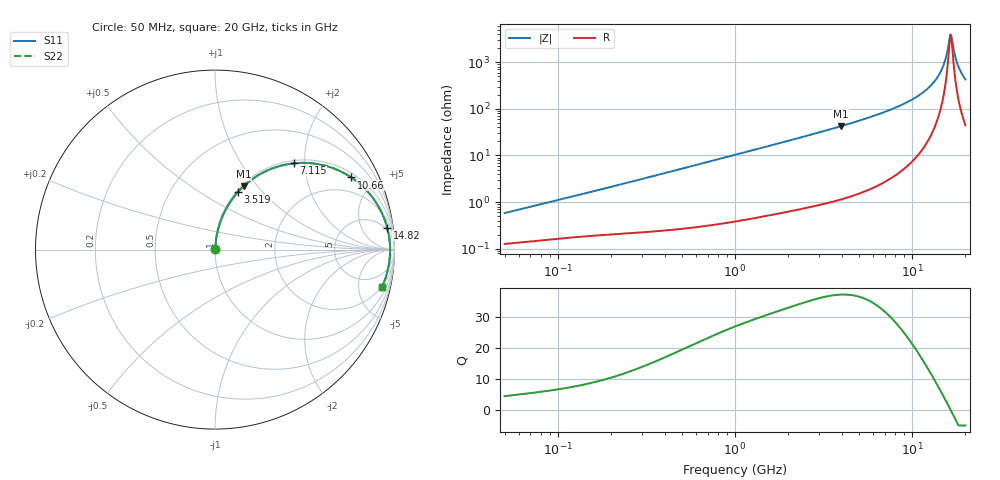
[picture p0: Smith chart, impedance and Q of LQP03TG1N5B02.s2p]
!Murata Part Number: LQP03TG1N5B02
!These Parameters are Measured in Series Mode Connection
!  o--[Z]--o
!Port1  Port2
!  o-------o
!Freq. Start=50[MHz] Stop=20[GHz], 401[Steps]
# Hz S RI R 50
!Freq.(Hz) S11(Real) S11(Imag) S21(Real) S21(Imag) S12(Real) S12(Imag) S22(Real) S22(Imag)
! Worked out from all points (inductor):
!   401 points, 50 MHz to 20 GHz, reference 50 ohm
!   read as one part in series: L = 1.78 nH near 51.52 MHz
!   highest Q = 37.3 at 3.967 GHz (marker M1), where L = 1.71 nH
!   self-resonance near 16.46 GHz
!   S11 on the Smith chart (normalised r, x): 50 MHz: 1.00, +0.01; 3.519 GHz: 1.02, +0.75; 7.115 GHz: 1.06, +1.76; 10.66 GHz: 1.19, +3.67; 14.82 GHz: 4, +15; 20 GHz: 1.89, -8.55
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5e7  0.0013 0.00565  0.9987 -0.00565  0.9987 -0.00565  0.0013 0.00565
1.364002e8  0.00203 0.0146  0.998 -0.0146  0.998 -0.0146  0.00203 0.0146
3.721004e8  0.00388 0.0386  0.9961 -0.0386  0.9961 -0.0386  0.00388 0.0386
1e9  0.0142 0.1013  0.9858 -0.1013  0.9858 -0.1013  0.0142 0.1013
2.728004e9  0.081 0.2591  0.919 -0.2591  0.919 -0.2591  0.081 0.2591
3.519108e9  0.1285 0.3215  0.8715 -0.3215  0.8715 -0.3215  0.1285 0.3215
3.967106e9  0.1597 0.3532  0.8403 -0.3532  0.8403 -0.3532  0.1597 0.3532
5.352748e9  0.2721 0.4314  0.7279 -0.4314  0.7279 -0.4314  0.2721 0.4314
7.114996e9  0.4379 0.4805  0.5621 -0.4805  0.5621 -0.4805  0.4379 0.4805
7.442007e9  0.4698 0.4829  0.5302 -0.4829  0.5302 -0.4829  0.4698 0.4829
1.066139e10  0.7596 0.4019  0.2404 -0.4019  0.2404 -0.4019  0.7596 0.4019
1.295331e10  0.8995 0.2592  0.1005 -0.2592  0.1005 -0.2592  0.8995 0.2592
1.396067e10  0.9377 0.1862  0.0623 -0.1862  0.0623 -0.1862  0.9377 0.1862
1.482269e10  0.9595 0.1225  0.0405 -0.1225  0.0405 -0.1225  0.9595 0.1225
1.550395e10  0.9699 0.0725  0.0301 -0.0725  0.0301 -0.0725  0.9699 0.0725
1.621653e10  0.9751 0.0214  0.0249 -0.0214  0.0249 -0.0214  0.9751 0.0214
1.646126e10  0.9757 0.00424  0.0243 -0.00424  0.0243 -0.00424  0.9757 0.00424
1.696185e10  0.9749 -0.0301  0.0251 0.0301  0.0251 0.0301  0.9749 -0.0301
1.774144e10  0.9692 -0.0812  0.0308 0.0812  0.0308 0.0812  0.9692 -0.0812
1.828096e10  0.9625 -0.1146  0.0375 0.1146  0.0375 0.1146  0.9625 -0.1146
1.912117e10  0.9482 -0.1634  0.0518 0.1634  0.0518 0.1634  0.9482 -0.1634
2e10  0.9291 -0.2099  0.0709 0.2099  0.0709 0.2099  0.9291 -0.2099
